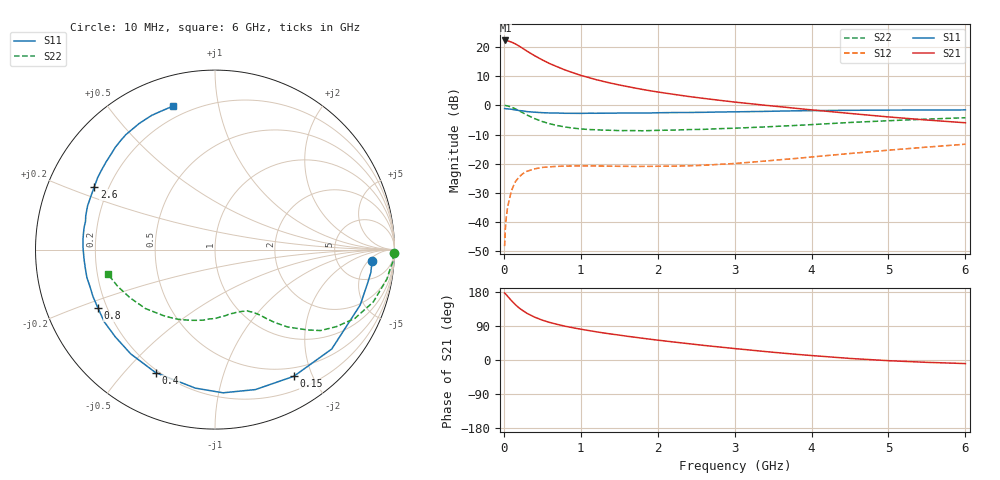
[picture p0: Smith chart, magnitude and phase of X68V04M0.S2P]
! SIEMENS Small Signal Semiconductors
! BFP193W
! Si NPN RF Bipolar Junction Transistor in SOT343
! VCE = 8 V  IC = 4 mA
! Common Emitter S-Parameters:  April 1994
# GHz  S  MA  R  50
!  f  S11  S21  S12  S22
! GHz  MAG  ANG  MAG  ANG  MAG  ANG  MAG  ANG
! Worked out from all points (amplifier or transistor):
!   40 points, 10 MHz to 6 GHz, reference 50 ohm
!   highest |S21| = 22.2 dB at 20 MHz (marker M1)
!   |S21| within 3 dB of that: start of sweep to 263.2 MHz
!   unconditionally stable (mu >= 1): 1.823 GHz to 4.449 GHz
!   at 200 MHz: K = 0.12, MSG = 22.3 dB, |S12| = -24.5 dB
!   at 1.5 GHz: K = 0.84, MSG = 13.9 dB, |S12| = -20.9 dB
!   at 6 GHz: K = 0.92, MSG = 3.7 dB, |S12| = -13.3 dB
!   S11 on the Smith chart (normalised r, x): 10 MHz: 12, -6; 150 MHz: 0.38, -1.74; 400 MHz: 0.19, -0.61; 800 MHz: 0.17, -0.23; 2.6 GHz: 0.15, +0.24; 6 GHz: 0.14, +0.74
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0.01  0.8776 -4.1  12.77 176.6  0.0039 87.7  0.9953 -1.2
0.02  0.8776 -8.4  12.82 175.1  0.0078 84.1  0.9926 -4.1
0.05  0.8658 -20.9  12.66 167.9  0.0185 78.5  0.9721 -9.7
0.1  0.8543 -40.4  12.01 156.5  0.0351 68.9  0.9288 -18.3
0.15  0.8314 -58.1  11.21 146.0  0.0494 60.1  0.8683 -26.2
0.2  0.8117 -73.9  10.23 137.1  0.0598 52.8  0.8021 -32.3
0.25  0.7992 -86.8  9.317 129.9  0.0682 46.4  0.741 -37.5
0.3  0.7794 -98.1  8.439 123.3  0.0743 41.7  0.6823 -41.0
0.4  0.7613 -115.7  7.037 113.1  0.0819 33.7  0.5914 -46.8
0.5  0.7471 -128.9  5.965 105.2  0.0865 29.0  0.5276 -50.5
0.6  0.7382 -138.8  5.132 98.9  0.0887 25.1  0.4812 -53.2
0.7  0.7367 -146.9  4.519 93.7  0.0904 22.9  0.4482 -55.1
0.8  0.7289 -153.4  3.994 89.0  0.0912 20.8  0.4247 -57.1
1.1  0.7305 -167.7  2.985 77.8  0.0917 18.0  0.385 -62.4
1.3  0.7313 -175.4  2.543 71.3  0.0914 17.6  0.3757 -66.3
1.6  0.7376 175.6  2.096 62.7  0.0905 18.5  0.3693 -72.2
2.2  0.7506 161.0  1.543 47.7  0.091 23.9  0.3761 -85.4
2.6  0.7579 152.5  1.31 38.5  0.0942 28.9  0.3875 -94.7
3.2  0.7792 141.1  1.065 26.3  0.106 35.5  0.4157 -108.6
4.5  0.8199 121.0  0.725 4.1  0.1497 41.4  0.5078 -139.7
5.5  0.828 110.9  0.559 -6.2  0.1926 39.1  0.5795 -159.3
6  0.8331 106.2  0.502 -9.4  0.2159 37.1  0.6123 -167.1
